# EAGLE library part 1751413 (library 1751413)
PCB terminal block, 3.5mm pitch, 2 level Source: Datasheet
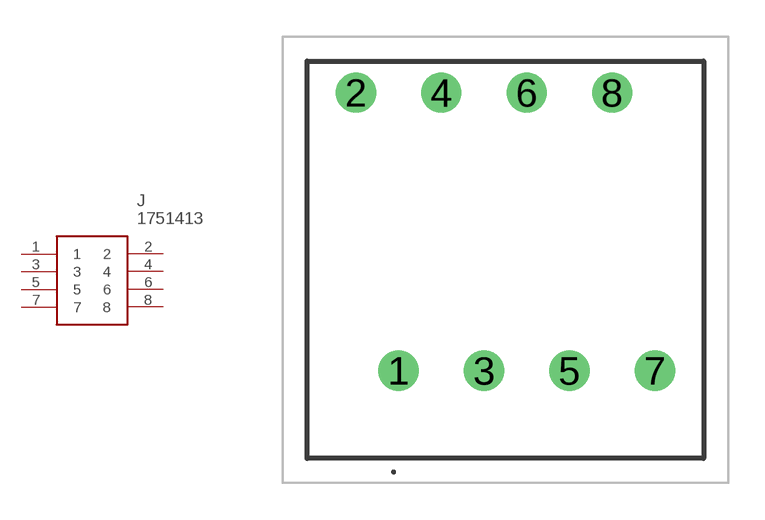
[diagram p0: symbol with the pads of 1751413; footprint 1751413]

Designator prefix J

## 1751413 (Arrow_Part_Number: 1751413; Arrow_Price-Stock: https://www.arrow.com/en/products/1751413/phoenix-contact?region=nac; Description: PCB terminal block, 3.5mm pitch, 2 level; Height: 16.35mm; Manufacturer_Name: Phoenix Contact; Manufacturer_Part_Number: 1751413; Mouser_Part_Number: 651-1751413; Mouser_Price-Stock: https://www.mouser.co.uk/ProductDetail/Phoenix-Contact/1751413?qs=IooffJMZQA61yzSPaR8Rbw%3D%3D)  [1751413]
1  1
2  2
3  3
4  4
5  5
6  6
7  7
8  8

## Footprint 1751413 (pad centres in mm)
1751413-1
drill 1.1 pad 1.65: 1 0,0; 2 -1.75,11.4; 3 3.5,0; 4 1.75,11.4; 5 7,0; 6 5.25,11.4; 7 10.5,0; 8 8.75,11.4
